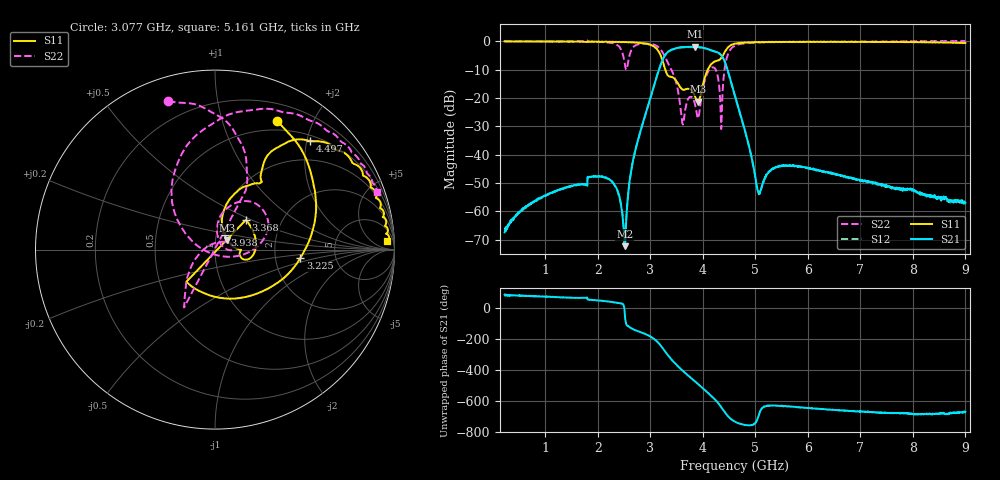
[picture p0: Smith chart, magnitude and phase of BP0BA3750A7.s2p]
!Agilent Technologies,E8358A,US41080443,A.07.50.56
!Agilent E8358A: A.07.50.56
!Date: Friday, December 15, 2017 21:15:24
!Correction: S11(Full 2 Port(1,2))
!S21(Full 2 Port(1,2))
!S12(Full 2 Port(1,2))
!S22(Full 2 Port(1,2))
!S2P File: Measurements: S11, S21, S12, S22:
# Hz S  dB  R 50
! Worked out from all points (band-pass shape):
!   1601 points, 225 MHz to 9 GHz, reference 50 ohm
!   highest |S21| = -1.97 dB at 3.856 GHz (marker M1); lowest = -72.3 dB at 2.512 GHz (marker M2)
!   |S21| within 3 dB of the highest: 3.279 GHz to 4.354 GHz (1.076 GHz wide, 28.2 % of centre)
!   lowest |S11| = -21.3 dB at 3.91 GHz (marker M3), VSWR 1.19, Z = 57.1 + j5.94 ohm
!   |S11| at or under -10 dB: 3.285 GHz to 4.095 GHz (810.3 MHz wide, 22 % of centre)
!   |S22| runs from -31.0 to 0.3 dB; largest |S21 - S12| = 0.011
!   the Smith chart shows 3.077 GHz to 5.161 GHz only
!   S11 on the Smith chart (normalised r, x): 3.077 GHz: 0.39, +1.52; 3.225 GHz: 2.78, -0.35; 3.368 GHz: 1.32, +0.46; 3.938 GHz: 1.10, +0.18; 4.497 GHz: 0.60, +2.06; 5.161 GHz: 20, +24
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2.25e8  -0.05 176.8  -67.38 84.3  -66.70 79.7  0.00 175.5
1.689328e9  -0.14 149.0  -50.41 63.5  -50.49 63.3  0.05 160.8
2.320031e9  -0.30 140.9  -50.72 34.6  -50.86 35.3  -0.91 101.1
2.511984e9  -0.37 132.5  -72.27 -33.8  -70.98 -28.9  -7.76 7.7
2.692969e9  -0.46 121.2  -40.19 -141.2  -40.19 -141.0  -1.77 170.0
3.076875e9  -1.98 64.2  -15.28 157.8  -15.32 157.9  -1.25 107.5
3.153656e9  -3.51 35.4  -10.60 134.2  -10.68 134.1  -2.11 93.6
3.224953e9  -6.42 -5.9  -6.90 105.1  -7.01 105.0  -3.70 79.8
3.367547e9  -12.45 43.9  -3.34 40.6  -3.43 40.8  -8.74 -118.1
3.614344e9  -17.04 -11.9  -2.08 -45.0  -2.18 -44.9  -29.13 122.6
3.855656e9  -19.63 8.6  -1.97 -115.4  -2.10 -115.5  -22.67 -0.9
3.9105e9  -21.31 36.9  -2.03 -131.4  -2.12 -131.4  -27.18 38.1
3.937922e9  -20.37 56.2  -2.07 -139.6  -2.17 -139.5  -24.56 69.7
4.272469e9  -6.84 55.5  -3.87 113.9  -3.98 114.0  -11.40 10.5
4.354734e9  -5.78 59.5  -4.98 77.8  -5.09 78.0  -29.83 -142.7
4.497328e9  -1.89 48.9  -11.78 14.7  -11.83 14.7  -3.76 98.9
4.6125e9  -0.84 34.3  -19.28 -13.8  -19.37 -13.4  -1.54 69.5
5.045766e9  -0.33 7.6  -52.68 8.9  -52.76 8.6  -0.44 26.2
5.160938e9  -0.36 2.8  -49.19 84.0  -49.05 81.6  -0.39 19.6
6.076828e9  -0.27 -22.7  -45.18 73.8  -45.16 72.9  -0.28 -16.3
7.541156e9  -0.23 -52.2  -51.14 42.5  -51.40 42.3  -0.11 -48.9
9e9  -0.61 -99.0  -57.02 50.4  -57.56 50.2  0.09 -43.4
